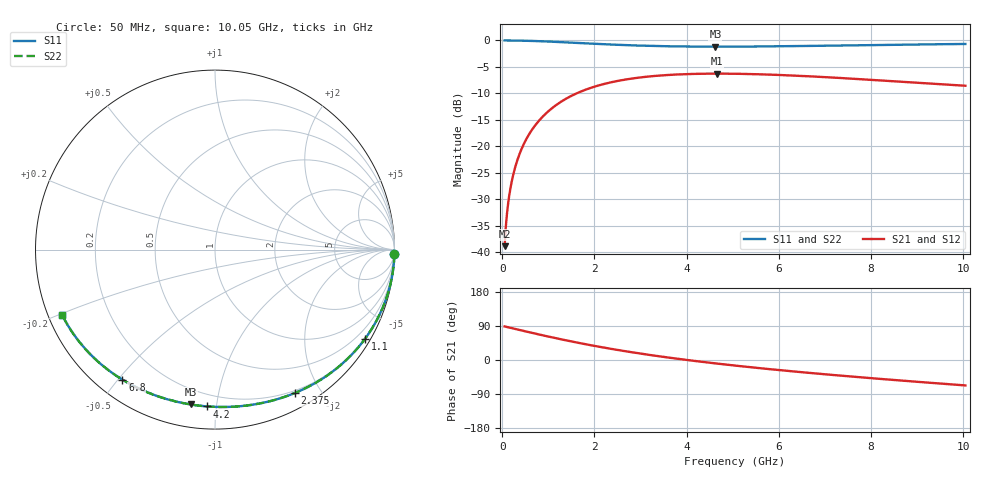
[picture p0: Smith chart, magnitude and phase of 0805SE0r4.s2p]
! AVX Thin Film Operation		Date: August 2001
! Description: Accu-P® Series, Thin Film, SMD, RF Capacitor
! Part Number: 08051J0R4ABT
! 50 MHz  -  10.05 GHz
! Serial Measurements
# mhz S db R 50
!	S11		S21		S12		S22
!	dB	Phase	dB	Phase	dB	Phase	dB	Phase
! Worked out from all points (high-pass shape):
!   401 points, 50 MHz to 10.05 GHz, reference 50 ohm
!   highest |S21| = -6.26 dB at 4.65 GHz (marker M1); lowest = -38.8 dB at 50 MHz (marker M2)
!   |S21| within 3 dB of the highest: 1.817 GHz to end of sweep
!   lowest |S11| = -1.2 dB at 4.625 GHz (marker M3), VSWR 14.81, Z = 5.83 - j42.4 ohm
!   |S11| at or under -10 dB: nowhere
!   |S22| runs from -1.2 to 0.0 dB; largest |S21 - S12| = 5.4e-05
!   S11 on the Smith chart (normalised r, x): 50 MHz: 0, -79; 1.1 GHz: 0.20, -3.62; 2.375 GHz: 0.17, -1.69; 4.2 GHz: 0.13, -0.94; 6.8 GHz: 0.07, -0.51; 10.05 GHz: 0.04, -0.20
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50  -0.00 -1.4  -38.83 88.6  -38.83 88.6  -0.00 -1.4
75  -0.00 -2.2  -35.31 87.9  -35.31 87.9  -0.00 -2.2
150  -0.01 -4.3  -29.30 85.7  -29.30 85.7  -0.01 -4.3
200  -0.01 -5.8  -26.81 84.2  -26.81 84.2  -0.01 -5.8
275  -0.02 -7.9  -24.06 82.1  -24.06 82.1  -0.02 -7.9
375  -0.03 -10.8  -21.41 79.2  -21.41 79.2  -0.03 -10.8
500  -0.06 -14.3  -18.97 75.6  -18.97 75.6  -0.06 -14.4
675  -0.10 -19.3  -16.48 70.7  -16.48 70.7  -0.10 -19.3
875  -0.16 -24.8  -14.39 65.2  -14.39 65.2  -0.16 -24.8
1100  -0.24 -30.8  -12.64 59.2  -12.64 59.2  -0.24 -30.8
1725  -0.51 -46.4  -9.57 43.5  -9.57 43.5  -0.51 -46.5
2375  -0.78 -60.8  -7.87 29.1  -7.87 29.1  -0.78 -60.9
2850  -0.93 -70.2  -7.14 19.7  -7.14 19.7  -0.93 -70.3
3400  -1.06 -80.1  -6.63 9.9  -6.63 9.9  -1.06 -80.1
4200  -1.16 -92.8  -6.31 -2.8  -6.31 -2.8  -1.16 -92.8
4625  -1.18 -98.9  -6.26 -9.0  -6.26 -9.0  -1.18 -98.9
4650  -1.18 -99.3  -6.26 -9.3  -6.26 -9.3  -1.18 -99.3
5050  -1.17 -104.7  -6.29 -14.7  -6.29 -14.7  -1.17 -104.7
6725  -1.03 -124.6  -6.79 -34.7  -6.79 -34.7  -1.03 -124.7
6800  -1.02 -125.4  -6.83 -35.5  -6.83 -35.5  -1.02 -125.5
8400  -0.83 -141.7  -7.65 -51.8  -7.65 -51.8  -0.83 -141.7
10050  -0.67 -156.9  -8.54 -67.1  -8.54 -67.1  -0.67 -157.0
